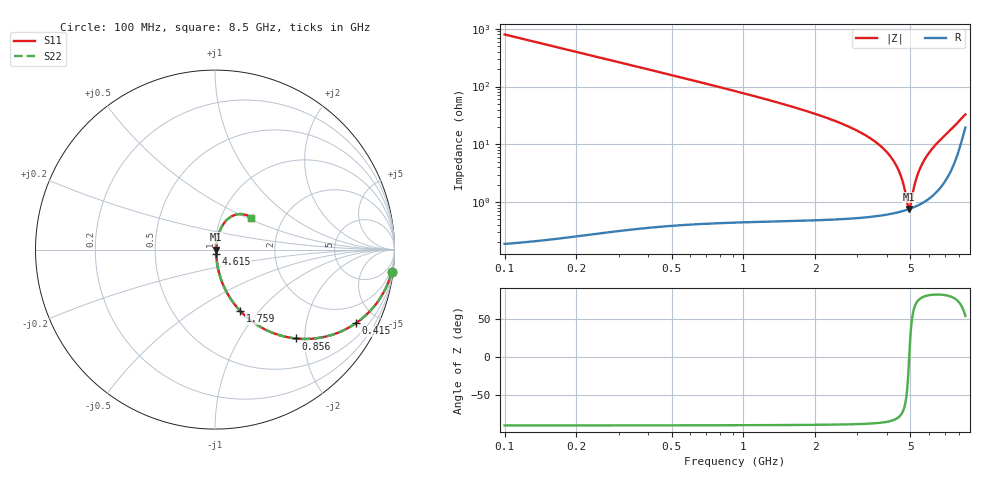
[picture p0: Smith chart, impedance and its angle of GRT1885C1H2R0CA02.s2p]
!Murata Part Number: GRT1885C1H2R0CA02
!These Parameters are Measured in Series Mode Connection
!Data Generated on Jun 19, 2026
!  o--ll--o
!Port1  Port2
!  o------o
!Operation Temp=25[degC], DC Bias Voltage=0[V]
!Freq. Start=100[MHz] Stop=9[GHz] 401[Steps]
# Hz S RI R 50
!Freq.(Hz) S11(Real) S11(Imag) S21(Real) S21(Imag) S12(Real) S12(Imag) S22(Real) S22(Imag)
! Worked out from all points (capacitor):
!   401 points, 100 MHz to 8.5 GHz, reference 50 ohm
!   read as one part in series: C = 2 pF near 142 MHz
!   lowest |Z| = 760 mohm at 4.951 GHz (marker M1)
!   series resonance near 4.946 GHz, so ESL is about 520 pH
!   S11 on the Smith chart (normalised r, x): 100 MHz: 1, -16; 415 MHz: 1.01, -3.81; 856 MHz: 1.01, -1.80; 1.759 GHz: 1.01, -0.80; 4.615 GHz: 1.01, -0.05; 8.5 GHz: 1.39, +0.53
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1e8  0.9844 -0.1238  0.0156 0.1238  0.0156 0.1238  0.9844 -0.1238
2.47e8  0.9115 -0.2836  0.0885 0.2836  0.0885 0.2836  0.9115 -0.2836
4.15e8  0.7832 -0.4111  0.2168 0.4111  0.2168 0.4111  0.7832 -0.4111
6.04e8  0.627 -0.482  0.373 0.482  0.373 0.482  0.627 -0.482
8.56e8  0.4491 -0.495  0.5509 0.495  0.5509 0.495  0.4491 -0.495
1.15e9  0.302 -0.4557  0.698 0.4557  0.698 0.4557  0.302 -0.4557
1.507e9  0.1902 -0.3877  0.8098 0.3877  0.8098 0.3877  0.1902 -0.3877
1.759e9  0.1394 -0.3405  0.8606 0.3405  0.8606 0.3405  0.1394 -0.3405
2.914e9  0.0367 -0.1742  0.9633 0.1742  0.9633 0.1742  0.0367 -0.1742
3.754e9  0.0142 -0.0912  0.9858 0.0912  0.9858 0.0912  0.0142 -0.0912
4.3e9  0.00861 -0.0468  0.9914 0.0468  0.9914 0.0468  0.00861 -0.0468
4.615e9  0.00743 -0.0233  0.9926 0.0233  0.9926 0.0233  0.00743 -0.0233
4.888e9  0.00742 -0.00398  0.9926 0.00398  0.9926 0.00398  0.00742 -0.00398
4.951e9  0.00754 0.000378  0.9925 -0.000378  0.9925 -0.000378  0.00754 0.000378
4.993e9  0.00764 0.00326  0.9924 -0.00326  0.9924 -0.00326  0.00764 0.00326
5.161e9  0.00826 0.0147  0.9917 -0.0147  0.9917 -0.0147  0.00826 0.0147
5.308e9  0.00906 0.0245  0.9909 -0.0245  0.9909 -0.0245  0.00906 0.0245
5.707e9  0.0125 0.0505  0.9875 -0.0505  0.9875 -0.0505  0.0125 0.0505
6.274e9  0.021 0.0868  0.979 -0.0868  0.979 -0.0868  0.021 0.0868
7.114e9  0.0461 0.1417  0.9539 -0.1417  0.9539 -0.1417  0.0461 0.1417
8.038e9  0.1231 0.1963  0.8769 -0.1963  0.8769 -0.1963  0.1231 0.1963
8.5e9  0.2023 0.1764  0.7977 -0.1764  0.7977 -0.1764  0.2023 0.1764
